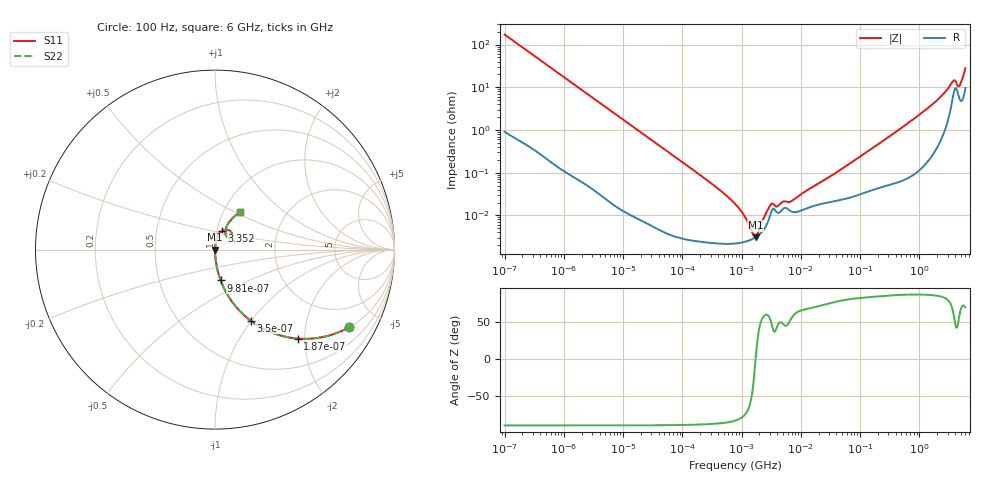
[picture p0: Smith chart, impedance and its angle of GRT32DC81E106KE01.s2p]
!Murata Part Number: GRT32DC81E106KE01
!These Parameters are Measured in Series Mode Connection
!Data Generated on Jun 19, 2026
!  o--ll--o
!Port1  Port2
!  o------o
!Operation Temp=25[degC], DC Bias Voltage=0[V]
!Freq. Start=100[Hz] Stop=6[GHz] 401[Steps]
# Hz S RI R 50
!Freq.(Hz) S11(Real) S11(Imag) S21(Real) S21(Imag) S12(Real) S12(Imag) S22(Real) S22(Imag)
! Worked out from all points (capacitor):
!   401 points, 100 Hz to 6 GHz, reference 50 ohm
!   read as one part in series: C = 9.21 uF near 109 Hz
!   lowest |Z| = 3.07 mohm at 1.734 MHz (marker M1)
!   series resonance near 1.725 MHz, so ESL is about 920 pH
!   S11 on the Smith chart (normalised r, x): 100 Hz: 1.02, -3.45; 187 Hz: 1.01, -1.85; 350 Hz: 1.01, -0.99; 981 Hz: 1.00, -0.35; 3.352 GHz: 1.06, +0.22; 6 GHz: 1.19, +0.53
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100  0.7475 -0.4318  0.2525 0.4318  0.2525 0.4318  0.7475 -0.4318
187  0.4608 -0.4956  0.5392 0.4956  0.5392 0.4956  0.4608 -0.4956
350  0.1983 -0.3956  0.8017 0.3956  0.8017 0.3956  0.1983 -0.3956
981  0.0315 -0.1717  0.9685 0.1717  0.9685 0.1717  0.0315 -0.1717
2008  0.00809 -0.0862  0.9919 0.0862  0.9919 0.0862  0.00809 -0.0862
40335  6.5e-05 -0.00438  0.9999 0.00438  0.9999 0.00438  6.5e-05 -0.00438
330837  2.26e-05 -0.000519  1 0.000519  1 0.000519  2.26e-05 -0.000519
774597  2.19e-05 -0.000186  1 0.000186  1 0.000186  2.19e-05 -0.000186
1159002  2.41e-05 -8.61e-05  1 8.61e-05  1 8.61e-05  2.41e-05 -8.61e-05
1734173  3.07e-05 1.2e-06  1 -1.2e-06  1 -1.2e-06  3.07e-05 1.2e-06
2372521  4.64e-05 7.42e-05  1 -7.42e-05  1 -7.42e-05  4.64e-05 7.42e-05
3245845  0.000131 0.000136  0.9999 -0.000136  0.9999 -0.000136  0.000131 0.000136
4060267  0.000115 0.000117  0.9999 -0.000117  0.9999 -0.000117  0.000115 0.000117
5079039  0.000145 0.000155  0.9999 -0.000155  0.9999 -0.000155  0.000145 0.000155
6644369  0.000127 0.000166  0.9999 -0.000166  0.9999 -0.000166  0.000127 0.000166
1.555665e7  0.000162 0.000427  0.9998 -0.000427  0.9998 -0.000427  0.000162 0.000427
3.124326e8  0.000563 0.00703  0.9994 -0.00703  0.9994 -0.00703  0.000563 0.00703
1.637704e9  0.00399 0.0389  0.996 -0.0389  0.996 -0.0389  0.00399 0.0389
3.352442e9  0.0394 0.1026  0.9606 -0.1026  0.9606 -0.1026  0.0394 0.1026
3.8344e9  0.0829 0.1063  0.9171 -0.1063  0.9171 -0.1063  0.0829 0.1063
4.796499e9  0.058 0.0854  0.942 -0.0854  0.942 -0.0854  0.058 0.0854
6e9  0.1376 0.2076  0.8624 -0.2076  0.8624 -0.2076  0.1376 0.2076
